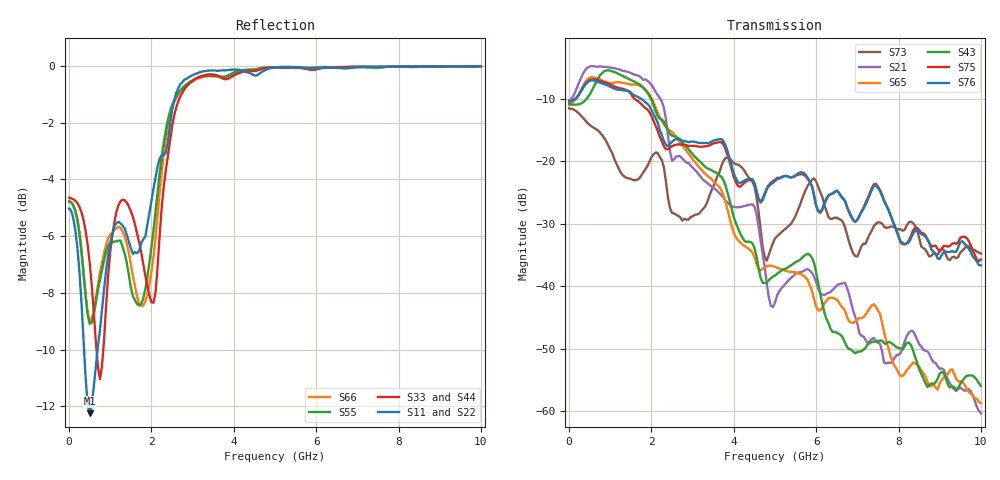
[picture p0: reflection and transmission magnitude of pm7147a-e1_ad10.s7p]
# GHz S DB R 50
! S-Parameters data
! Freq  dbS11  angS11  dbS12  angS12  dbS13  angS13  dbS14  angS14
!  dbS15  angS15  dbS16  angS16  dbS17  angS17  dbS21  angS21
!  dbS22  angS22  dbS23  angS23  dbS24  angS24  dbS25  angS25
!  dbS26  angS26  dbS27  angS27  dbS31  angS31  dbS32  angS32
!  dbS33  angS33  dbS34  angS34  dbS35  angS35  dbS36  angS36
!  dbS37  angS37  dbS41  angS41  dbS42  angS42  dbS43  angS43
!  dbS44  angS44  dbS45  angS45  dbS46  angS46  dbS47  angS47
!  dbS51  angS51  dbS52  angS52  dbS53  angS53  dbS54  angS54
!  dbS55  angS55  dbS56  angS56  dbS57  angS57  dbS61  angS61
!  dbS62  angS62  dbS63  angS63  dbS64  angS64  dbS65  angS65
!  dbS66  angS66  dbS67  angS67  dbS71  angS71  dbS72  angS72
!  dbS73  angS73  dbS74  angS74  dbS75  angS75  dbS76  angS76
!  dbS77  angS77
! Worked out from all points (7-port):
!   279 points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, 1 Hz to 10 GHz, reference 50 ohm
!   strongest paths, dB at 1 Hz, 7.943 MHz, 3.05 GHz, 6.55 GHz, 10 GHz:
!     S76: -10.4, -10.4, -16.9, -25.1, -36.7
!     S75: -10.4, -10.4, -17.6, -25.1, -35.7
!     S43: -11.0, -11.0, -19.3, -47.6, -56.0
!     S65: -10.7, -10.7, -20.1, -42.6, -58.7
!     S21: -10.3, -10.3, -21.4, -39.7, -60.3
!     S73: -11.6, -11.6, -28.6, -29.2, -34.8
!   lowest |S11| = -12.2 dB at 500 MHz (marker M1), VSWR 1.65, Z = 30.4 + j0.162 ohm
!   |S11| at or under -10 dB: 363.5 MHz to 691.7 MHz (328.2 MHz wide, 62.2 % of centre)
